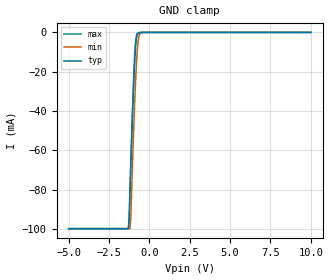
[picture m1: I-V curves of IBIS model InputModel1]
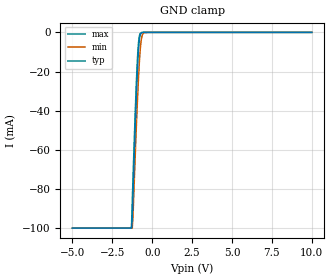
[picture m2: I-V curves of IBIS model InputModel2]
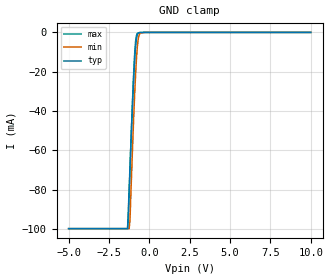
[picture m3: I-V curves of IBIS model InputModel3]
[IBIS Ver]   2.1
[File name]   e_002bv5.ibs   | e_= TSOP, f002bv= abbr chip name, 5= 5V Vcc
[File Rev]   2.00
[Date]   28-February-96
[Source]   File generated from lab measurements at Intel Corporation
[Notes]   Rev 2.00 All data was replaced by actual measurements
   performed in a lab.
[Disclaimer] INTEL DEVELOPER'S SOFTWARE LICENSE AGREEMENT
| BY USING THIS SOFTWARE, YOU ARE AGREEING TO BE BOUND
| BY THE TERMS OF THIS AGREEMENT.  DO NOT USE THE SOFTWARE
| UNTIL YOU HAVE CAREFULLY READ AND AGREED TO THE FOLLOWING
| TERMS AND CONDITIONS.  IF YOU DO NOT AGREE TO THE TERMS
| OF THIS AGREEMENT, PROMPTLY RETURN THE SOFTWARE PACKAGE
| AND ANY ACCOMPANYING ITEMS.
| IF YOU USE THIS SOFTWARE, YOU WILL BE BOUND BY THE TERMS
| OF THIS AGREEMENT
| LICENSE: Intel Corporation ("Intel") grants you the non-exclusive right
| to use the enclosed software program ("Software").  You will not use,
| copy, modify, rent, sell or transfer the Software or any portion
| thereof, except as provided in this Agreement.
| System OEM Developers may:
| 1.   Copy the Software for support, backup or archival purposes;
| 2.   Install, use, or distribute Intel owned Software in object code
|   only;
| 3.   Modify and/or use Software source code that Intel directly makes
|   available to you as an OEM Developer;
| 4.   Install, use, modify, distribute, and/or make or have made
|   derivatives ("Derivatives") of Intel owned Software under the
|   terms and conditions in this Agreement, ONLY if you are a System
|   OEM Developer and NOT an end-user.
| RESTRICTIONS:
| YOU WILL NOT:
| 1.   Copy the Software, in whole or in part, except as provided for
|   in this Agreement;
| 2.   Decompile or reverse engineer any Software provided in object
|   code format;
| 3.   Distribute any Software or Derivative code to any end-users,
|   unless approved by Intel in a prior writing.
| TRANSFER: You may transfer the Software to another OEM
| Developer if the receiving party agrees to the terms of this
| Agreement at the sole risk of any receiving party.
| OWNERSHIP AND COPYRIGHT OF SOFTWARE:
| Title to the Software and all copies thereof remain with Intel
| or its vendors.  The Software is copyrighted and is protected by
| United States and international copyright laws.  You will not
| remove the copyright notice from the Software.  You agree to
| prevent any unauthorized copying of the Software.
| DERIVATIVE WORK: OEM Developers that make or have made
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[Copyright]   Copyright 1996, Intel Corporation, All Rights Reserved
[Component]   E28F002BV   | 40-lead TSOP package, 28F002BV
[Manufacturer]  Intel   | Boot Block (tm)
|   | operating in 5V Vcc range
[Package]
|Variable   typ   min   max
|The following values apply for the leadframe.
R_pkg   135m   126m   144m
L_pkg   3.95nH   3.62nH   4.28nH
C_pkg   0.39pF   0.38pF   0.40pF
|*****************************Pin Definitions**********************************
[Pin]   signal_name   model_name   R_pin   L_pin   C_pin
 1   A16   InputModel2
 2   A15   InputModel3
 3   A14   InputModel3
 4   A13   InputModel3
 5   A12   InputModel3
 6   A11   InputModel3
 7   A09   InputModel3
 8   A08   InputModel3
 9   WE#   InputModel1
10   RP#   InputModel1
11   VPP   POWER
12   WP#   InputModel1
13   NC   InputModel3
14   A07   InputModel3
15   A06   InputModel3
16   A05   InputModel3
17   A04   InputModel3
18   A03   InputModel3
19   A02   InputModel3
20   A01   InputModel3
21   A00   InputModel2
22   CE#   InputModel1
23   GND   GND
24   OE#   InputModel1
25   DQ0   InputOutput
26   DQ1   InputOutput
27   DQ2   InputOutput
28   DQ3   InputOutput
29   NC   InputModel4
30   VCC   POWER
31   VCC   POWER
32   DQ4   InputOutput
33   DQ5   InputOutput
34   DQ6   InputOutput
35   DQ7   InputOutput
36   A10   InputModel3
37   NC   InputModel3
38   NC   InputModel4
39   GND   GND
40   A17   InputModel3
|***********************Input Model 4******************************
[Model]   InputModel4
Model_type   Input
|   Model for NC pins (Numbers 29 & 38).
Vinl = 0.8V
Vinh = 2.0V
|Variable   Typ   Min   Max
C_comp   5.61p   NA   7.6p
[Voltage Range]   5.0V   4.5V   5.5V
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| Models and submodels in the file (5): InputModel1 (Input), InputModel2 (Input), InputModel3 (Input), InputModel4 (Input), InputOutput (I/O)
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|*********************Input Model 1************************************
[Model]   InputModel1
Model_type   Input
|   Model for WE#, WP#, RP#, OE# & CE#.
Vinl = 0.8V
Vinh = 2.0V
|Variable   Typ   Min   Max
C_comp   5.61p   NA   7.6p
[Voltage Range]   5.0V   4.5V   5.5V
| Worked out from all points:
|   GND clamp passes 1 mA (typ) near -0.74 V on its own axis
[GND_clamp]
|Voltage  I(typ)   I(min)   I(max)
-5V       -99.85mA   -99.85mA   -99.85mA
-1.3V     -99.85mA   -99.85mA   -99.85mA
-1.25V    -93.26mA   -99.85mA   -95.79mA
-1.2V     -80.3mA    -99.85mA   -81.5mA
-1.15V    -67.6mA    -94.88mA   -67.39mA
-1V       -32.49mA   -56.57mA   -29.26mA
-900mV    -13.7mA    -33.97mA   -10.19mA
-850mV    -7.324mA   -24.38mA   -4.514mA
-750mV    -1.17mA    -9.368mA   -570.4uA
-650mV    -196.9uA   -2.246mA   -163.7uA
-500mV    -19.68uA   -149.2uA   0A
10V       0A         0A         0A
[Power_clamp]
| Input buffer circuits of this product do not intrinsically
| require a [Power_clamp] definition.  This zero current
| [Power_clamp] table is provided for the compatibility with
| some IBIS parsers.
|Voltage  I(typ)   I(min)   I(max)
-5V       0A         0A         0A
0V        0A         0A         0A
5V        0A         0A         0A
10V       0A         0A         0A
|*********************Input Model 2******************************
[Model]   InputModel2
Model_type   Input
|   Model for A[0] & A[16] pins.
Vinl = 0.8V
Vinh = 2.0V
|Variable   Typ   Min   Max
C_comp   5.61p   NA   7.6p
[Voltage Range]   5.0V   4.5V   5.5V
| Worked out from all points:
|   GND clamp passes 1 mA (typ) near -0.74 V on its own axis
[GND_clamp]
|Voltage  I(typ)   I(min)   I(max)
-5V       -99.85mA   -99.85mA   -99.85mA
-1.3V     -99.85mA   -99.85mA   -99.7mA
-1.25V    -95.1mA    -99.85mA   -86.57mA
-1.2V     -81.91mA   -93.12mA   -73.81mA
-1.05V    -44.51mA   -59.81mA   -37.94mA
-950mV    -22.91mA   -39.4mA    -17.7mA
-900mV    -14.12mA   -30.1mA    -9.812mA
-850mV    -7.485mA   -21.87mA   -4.492mA
-750mV    -1.181mA   -8.658mA   -581.8uA
-650mV    0A         -2.149mA   -166uA
-500mV    0A         -145.6uA   -18.8uA
10V       0A         0A         0A
[Power_clamp]
| Input buffer circuits of this product do not intrinsically
| require a [Power_clamp] definition.  This zero current
| [Power_clamp] table is provided for the compatibility with
| some IBIS parsers.
|Voltage  I(typ)   I(min)   I(max)
-5V       0A         0A         0A
0V        0A         0A         0A
5V        0A         0A         0A
10V       0A         0A         0A
|***********************Input Model 3******************************
[Model]   InputModel3
Model_type   Input
|   Model for A[15:1], A[17] & NC pin #13 & #37.
Vinl = 0.8V
Vinh = 2.0V
|Variable   Typ   Min   Max
C_comp   5.61p   NA   7.6p
[Voltage Range]   5.0V   4.5V   5.5V
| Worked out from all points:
|   GND clamp passes 1 mA (typ) near -0.74 V on its own axis
[GND_clamp]
|Voltage  I(typ)   I(min)   I(max)
-5V       -99.85mA   -99.86mA   -99.85mA
-1.35V    -99.85mA   -99.86mA   -99.85mA
-1.3V     -90.17mA   -99.86mA   -94.83mA
-1.25V    -79.25mA   -99.86mA   -82.83mA
-1.2V     -68.58mA   -95.57mA   -70.38mA
-1.05V    -38.07mA   -60.6mA    -36.34mA
-950mV    -20.19mA   -39.21mA   -17.09mA
-850mV    -7.009mA   -21.02mA   -4.405mA
-750mV    -1.188mA   -7.828mA   -577.2uA
-600mV    -101.4uA   -746.5uA   -94.18uA
-250mV    0A         0A         0A
10V       0A         0A         0A
[Power_clamp]
| Input buffer circuits of this product do not intrinsically
| require a [Power_clamp] definition.  This zero current
| [Power_clamp] table is provided for the compatibility with
| some IBIS parsers.
|Voltage  I(typ)   I(min)   I(max)
-5V       0A         0A         0A
0V        0A         0A         0A
5V        0A         0A         0A
10V       0A         0A         0A
